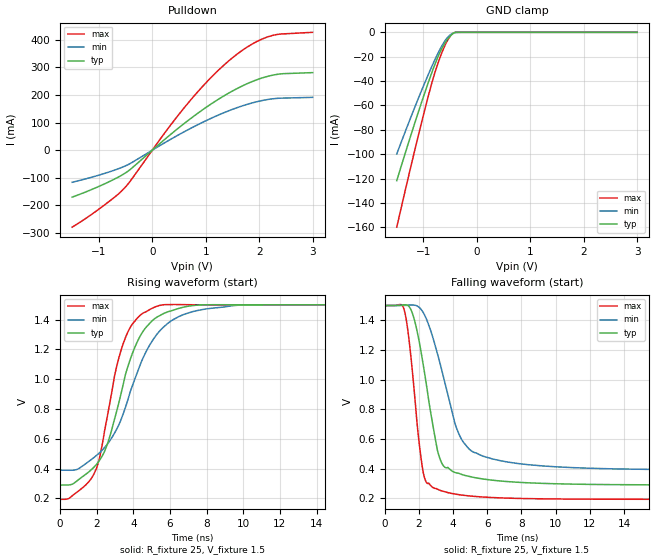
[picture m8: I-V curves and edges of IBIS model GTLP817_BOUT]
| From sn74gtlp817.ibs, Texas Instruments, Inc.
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[Model]   GTLP817_BOUT
Model_type  Open_drain
Vref =   1.5
Rref =   25
Cref =   30p
Vmeas =   1.0
| variable   typ   min   max
C_comp   3.98pF   3.39pF   4.39pF
| C_pulldown   4.66pF   3.42pF   7.11pF
| C_tri-state   3.98pF   3.39pF   4.39pF
[Temperature Range]   40   100   -40
| Ambient temperature   25   85   -40
[Voltage range]   1.5   1.5   1.5
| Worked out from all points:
|   slope of the pulldown table from 0 to 0.225 V, typ, clamps not added: 5.95 ohm
|   GND clamp passes 1 mA (typ) near -0.45 V on its own axis
|   rising waveform, R_fixture 25, V_fixture 1.5: 20-80 % time 1.76ns typ, 2.3ns min, 1.33ns max; typ from 0.29 V to 1.5 V
|   falling waveform, R_fixture 25, V_fixture 1.5: 20-80 % time 1.06ns typ, 1.6ns min, 693ps max; typ from 1.5 V to 0.29 V
[GND Clamp]
| GTLP817_BOUT
|   Voltage   I(typ)   I(min)   I(max)
-1.5V     -121.7mA   -99.72mA   -159.8mA
-1.295V   -92.63mA   -76.24mA   -121mA
-1.11V    -67.27mA   -55.72mA   -87.16mA
-945mV    -45.64mA   -38.21mA   -58.28mA
-825mV    -30.84mA   -26.19mA   -38.72mA
-715mV    -18.62mA   -16.03mA   -23.68mA
-625mV    -10.72mA   -8.841mA   -13.43mA
-535mV    -4.824mA   -3.591mA   -5.529mA
-455mV    -1.248mA   -851.3uA   -1.097mA
-415mV    -278.6uA   -180.1uA   -123.4uA
-360mV    -12.77uA   -26.08uA   -10.45uA
3V        478.1pA    2.154nA    3.61nA
[Pulldown]
| GTLP817_BOUT
|   Voltage   I(typ)   I(min)   I(max)
-1.5V     -170.1mA   -116.3mA   -278.9mA
-950mV    -127mA     -87.6mA    -206.5mA
-530mV    -85.79mA   -59.17mA   -139.1mA
-410mV    -69.46mA   -47.93mA   -111.4mA
285mV     47.64mA    32.86mA    76.11mA
660mV     106.1mA    73.17mA    168.4mA
1.1V      167.2mA    115.4mA    263.4mA
1.505V    214.9mA    148.2mA    335.4mA
1.86V     247.9mA    170.6mA    383.5mA
2.185V    268.7mA    184.3mA    412mA
2.405V    276.3mA    188.5mA    420.8mA
3V        281mA      191.3mA    427mA
[Ramp]
| GTLP817_BOUT
| variable   typ   min   max
dV/dt_r   0.73/1.80E-09   0.67/2.35E-09   0.78/1.38E-09
dV/dt_f   0.73/1.07E-09   0.67/1.70E-09   0.79/7.14E-10
R_load = 25
[Rising Waveform]
| GTLP817_BOUT
R_fixture =   25
C_fixture =   0
L_fixture =   0
V_fixture =   1.5
V_fixture_min = 1.5
V_fixture_max = 1.5
|   Time   V(typ)   V(min)   V(max)
0s        289.5mV    389.2mV    193.5mV
1.645ns   386.2mV    455.6mV    324.1mV
2.31ns    487.9mV    525.7mV    569mV
2.98ns    736.7mV    640.7mV    1.029V
3.545ns   1.022V     803.7mV    1.273V
4.305ns   1.275V     1.076V     1.423V
5.15ns    1.406V     1.279V     1.484V
6.685ns   1.483V     1.432V     1.501V
9.465ns   1.5V       1.495V     1.5V
24.99ns   1.5V       1.5V       1.5V
[Falling Waveform]
| GTLP817_BOUT
R_fixture =   25
C_fixture =   0
L_fixture =   0
V_fixture =   1.5
V_fixture_min = 1.5
V_fixture_max = 1.5
|   Time   V(typ)   V(min)   V(max)
0s        1.5V       1.5V       1.5V
1.15ns    1.505V     1.501V     1.466V
1.66ns    1.433V     1.503V     1.004V
2.23ns    1.115V     1.457V     387.8mV
2.875ns   654.3mV    1.261V     269.7mV
3.375ns   429.2mV    1.046V     249.2mV
4.32ns    369.5mV    639.2mV    225.4mV
5.77ns    330.4mV    483.9mV    209.1mV
10.94ns   296.3mV    407.7mV    195.3mV
24.99ns   289.8mV    390.1mV    193.7mV
